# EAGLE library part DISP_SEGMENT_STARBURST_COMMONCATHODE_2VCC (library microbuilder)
Starburst Segment Display - Common Cathode 2.3" Red Alphanumeric LED Display - BL-S230B-12
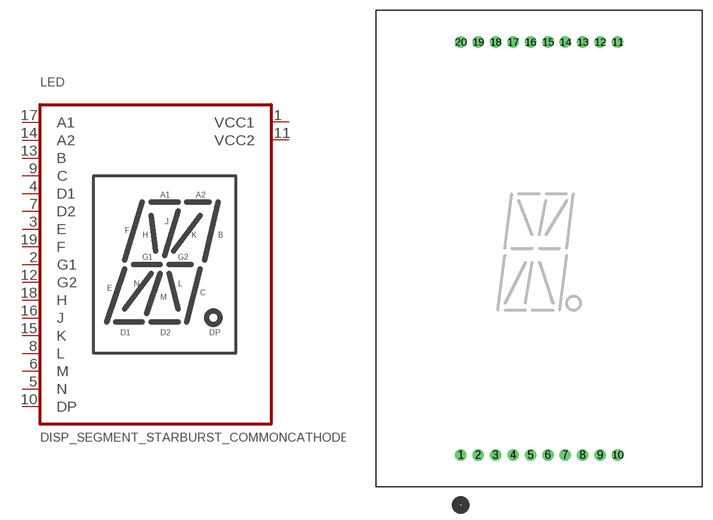
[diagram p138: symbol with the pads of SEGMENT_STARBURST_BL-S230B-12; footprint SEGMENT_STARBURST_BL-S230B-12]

Designator prefix LED

## DISP_SEGMENT_STARBURST_COMMONCATHODE_2VCCBLS230B12  [SEGMENT_STARBURST_BL-S230B-12]
1  VCC1  pwr
2  G1
3  E
4  D1
5  N
6  M
7  D2
8  L
9  C
10  DP
11  VCC2  pwr
12  G2
13  B
14  A2
15  K
16  J
17  A1
18  H
19  F

## Footprint SEGMENT_STARBURST_BL-S230B-12 (pad centres in mm)
drill 0.8 pad 1.676: 1 -11.43,-30.1; 2 -8.89,-30.1; 3 -6.35,-30.1; 4 -3.81,-30.1; 5 -1.27,-30.1; 6 1.27,-30.1; 7 3.81,-30.1; 8 6.35,-30.1; 9 8.89,-30.1; 10 11.43,-30.1; 11 11.43,30.1; 12 8.89,30.1; 13 6.35,30.1; 14 3.81,30.1; 15 1.27,30.1; 16 -1.27,30.1; 17 -3.81,30.1; 18 -6.35,30.1; 19 -8.89,30.1; 20 -11.43,30.1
